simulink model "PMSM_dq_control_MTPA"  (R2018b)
settings: Solver=VariableStepAuto  StartTime=0.0  StopTime=765  FixedStep=1e-5  RelTol=1e-8
InitFcn:
  | I_peak = 230
  | Ke_nom = 0.92
  | Ld_nom = 1.52e-3
  | Lq_nom = 1.54e-3
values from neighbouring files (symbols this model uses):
  B = 0    [Tesla_Initialization.m]    (also in PMSM_EV_init_v2.m; Leaf_Initialization.m)
  J = 0.3    [Tesla_Initialization.m]    (also in PMSM_EV_init_v2.m; Leaf_Initialization.m)
  P = 8    [Tesla_Initialization.m]    (also in PMSM_EV_init_v2.m; Iqbal Husain - Example12_1.m = V.*I; Leaf_Initialization.m)
  radius = 0.447    [Tesla_Initialization.m]    (also in PMSM_EV_init_v2.m = 0.3; Leaf_Initialization.m)
  ratio = 9    [Tesla_Initialization.m]    (also in PMSM_EV_init_v2.m; Leaf_Initialization.m)
  Rs = 0.046    [Tesla_Initialization.m]    (also in PMSM_EV_init_v2.m; Leaf_Initialization.m)
  Tesla_id_axis = [-8.764242E+02	-7.790438E+02	-6.816633E+02	-5.842828E+02	-4.869024E+02	-3.895219E+02	-2.921414E+02	-1.947609E+02	-9.738047E+01	+0.000000E+00]    [Tesla_Initialization.m]
  Tesla_iq_axis = [+0.000000E+00	+9.738047E+01	+1.947609E+02	+2.921414E+02	+3.895219E+02	+4.869024E+02	+5.842828E+02	+6.816633E+02	+7.790438E+02	+8.764242E+02]    [Tesla_Initialization.m]
  Tesla_Ld = [+8.821895E-05	+8.924938E-05	+9.139742E-05	+9.462732E-05	+1.042993E-04	+1.207302E-04	+1.435858E-04	+1.651379E-04	+1.771179E-04	+1.815302E-04    [Tesla_Initialization.m]
  Tesla_Lq = [+2.750008E-04	+2.848007E-04	+2.919706E-04	+2.981362E-04	+3.048757E-04	+3.200995E-04	+3.552424E-04	+3.955550E-04	+4.296280E-04	+4.500669E-04    [Tesla_Initialization.m]
  Tesla_phid = [-9.964313E-02	-8.749389E-02	-7.506085E-02	-6.231998E-02	-4.899731E-02	-3.359246E-02	-1.574417E-02	+5.955898E-03	+2.974036E-02	+5.474011E-02    [Tesla_Initialization.m]
  Tesla_phiq = [+1.577834E-05	+2.291095E-05	+1.626960E-05	+6.018524E-06	+7.523247E-06	+1.073346E-05	+2.148179E-05	+1.486713E-05	+9.491501E-06	-7.613491E-07    [Tesla_Initialization.m]
undefined symbols (not defined in the file or in its folder): A1, B766, HEV_Param
libraries: fl_lib x18, nesl_utility x9, sdl_lib x4

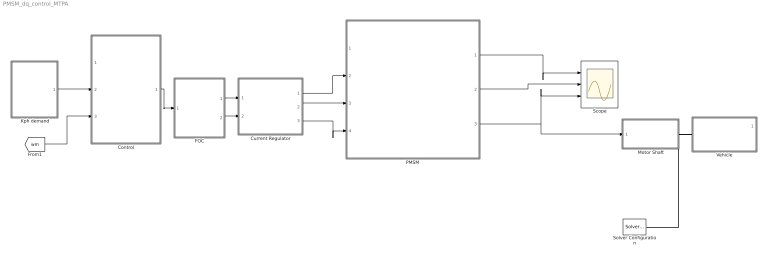
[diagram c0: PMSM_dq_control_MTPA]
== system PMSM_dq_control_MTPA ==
  Control : Subsystem
  Current Regulator : Subsystem
  FOC : Subsystem
  Kph demand : Subsystem
  Motor Shaft : Subsystem
  PMSM : Subsystem
  Scope : Scope  NumInputPorts=3
  Solver Configuration : nesl_utility/Solver Configuration  PhysicalDomain=network_engine_domain  SubClassName=solver  LeftPortType=input  RightPortType=generic  Tones=[]  Harmonics=[]  SimulateNoise=off  Profile=off  UseLocalSampling=off  EnableSwitchedLinearOptims=on  FrequencyDomain=off  UseCCode=off  RelTol=0.001  AbsTol=1e-06  MinStep=1e-09  ToWorkspace=off  RevertToSquareIcSolve=off  NumHomotopyIterations=100  PhasorMode=off  PhasorModeNumHarmonics=1  DoDC=off  ResidualTolerance=1e-09  UseLocalSolver=off  LocalSolverChoice=NE_BACKWARD_EULER_ADVANCER  LocalSolverSampleTime=0.001  DoFixedCost=off  MaxNonlinIter=3  MaxModeIter=2  LinearAlgebra=auto  EquationFormulation=NE_TIME_EF  DelaysMemoryBudget=1024  AutomaticFiltering=on  FilteringTimeConstant=0.001  PartitionStorageMethod=AS_NEEDED  PartitionMemoryBudget=1024
  Vehicle : Subsystem
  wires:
  Current Regulator/1(Va) -> PMSM/2(Va)
  Kph demand/1(Ref omega) -> Control/2(omega_ref)
  PMSM/3(Torque (Nm)) -> Motor Shaft/1(In1), Scope/3
  FOC/2(Id_ref) -> Current Regulator/2(id_ref)
  FOC/1(Iq_ref) -> Current Regulator/1(iq_ref)
  Current Regulator/2(Vb) -> PMSM/3(Vb)
  Current Regulator/3(Vc) -> PMSM/4(Vc)
  PMSM/1(iabc) -> Scope/1
  Control/1(Tref) -> FOC/1(Tref)
  [wm] -> Control/3(omega)
  PMSM/2(wm) -> Scope/2
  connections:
  Vehicle/LConn1 -- Solver Configuration/RConn1 -- Motor Shaft/RConn1

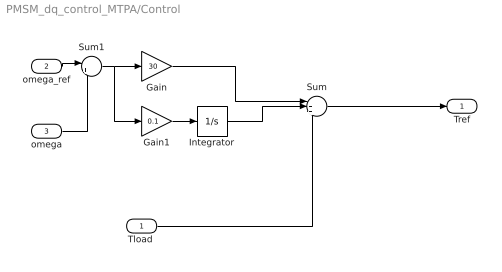
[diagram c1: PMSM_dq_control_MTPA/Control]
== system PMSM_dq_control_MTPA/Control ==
  "Tload " : Inport
  omega_ref : Inport  Port=2
  omega : Inport  Port=3
  Gain : Gain  Gain=30
  Gain1 : Gain  Gain=0.1
  Integrator : Integrator
  Sum : Sum  Inputs=|+++
  Sum1 : Sum  Inputs=|+-
  Tref : Outport
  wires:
  omega_ref/1 -> Sum1/1
  Sum1/1 -> Gain1/1, Gain/1
  omega/1 -> Sum1/2
  Gain1/1 -> Integrator/1
  "Tload "/1 -> Sum/3
  Integrator/1 -> Sum/2
  Gain/1 -> Sum/1
  Sum/1 -> Tref/1

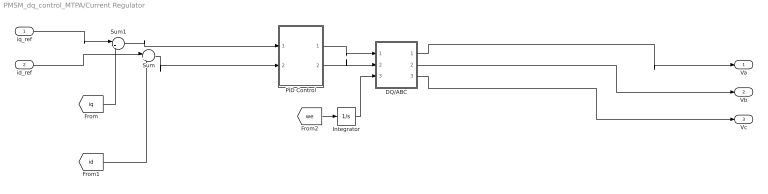
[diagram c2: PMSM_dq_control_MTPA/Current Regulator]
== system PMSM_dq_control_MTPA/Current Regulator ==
  iq_ref : Inport
  id_ref : Inport  Port=2
  DQ/ABC : Subsystem
  Integrator : Integrator
  PID Control : Subsystem
  Sum : Sum  Inputs=|+-
  Sum1 : Sum  Inputs=|+-
  Va : Outport
  Vb : Outport  Port=2
  Vc : Outport  Port=3
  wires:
  [iq] -> Sum1/2
  [id] -> Sum/2
  PID Control/1(Out1) -> DQ/ABC/1(Vq)
  Sum/1 -> PID Control/2(In3)
  PID Control/2(Out2) -> DQ/ABC/2(Vd)
  id_ref/1 -> Sum/1
  [we] -> Integrator/1
  iq_ref/1 -> Sum1/1
  Integrator/1 -> DQ/ABC/3(theta_rf)
  Sum1/1 -> PID Control/1(In1)
  DQ/ABC/1(Va) -> Va/1
  DQ/ABC/2("Vb ") -> Vb/1
  DQ/ABC/3("Vc ") -> Vc/1

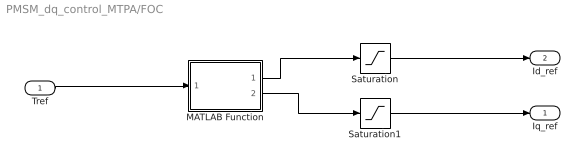
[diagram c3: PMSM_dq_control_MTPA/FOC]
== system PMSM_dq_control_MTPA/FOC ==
  Tref : Inport
  MATLAB Function : MATLAB Function  TreatAsAtomicUnit=on
  Saturation : Saturate  UpperLimit=230  LowerLimit=-230
  Saturation1 : Saturate  UpperLimit=230  LowerLimit=-230
  Iq_ref : Outport
  Id_ref : Outport  Port=2
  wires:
  MATLAB Function/2(iq) -> Saturation1/1
  Saturation/1 -> Id_ref/1
  Saturation1/1 -> Iq_ref/1
  MATLAB Function/1(id) -> Saturation/1
  Tref/1 -> MATLAB Function/1(Te)

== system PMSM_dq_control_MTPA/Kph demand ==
  From Spreadsheet4 : FromSpreadsheet  FileName=Highway_cycle.xlsx  Range=A1:B766  ExtrapolationBeforeFirstDataPoint=Hold first value
  Gain : Gain  Gain=1.6*5/18*ratio/radius
  Ref omega : Outport
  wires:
  From Spreadsheet4/1 -> Gain/1
  Gain/1 -> Ref omega/1

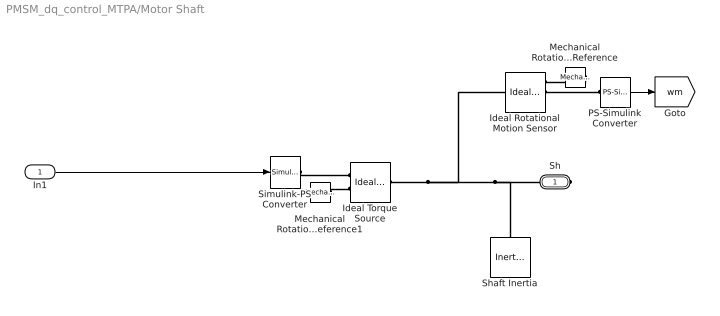
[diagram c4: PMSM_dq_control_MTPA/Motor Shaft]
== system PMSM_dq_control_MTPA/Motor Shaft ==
  In1 : Inport
  Ideal Rotational Motion Sensor : fl_lib/Mechanical/Mechanical Sensors/Ideal Rotational Motion Sensor  offset=0 rad
  Ideal Torque Source : fl_lib/Mechanical/Mechanical Sources/Ideal Torque Source
  Mechanical Rotational Reference : fl_lib/Mechanical/Rotational Elements/Mechanical Rotational Reference
  Mechanical Rotational Reference1 : fl_lib/Mechanical/Rotational Elements/Mechanical Rotational Reference
  PS-Simulink Converter : nesl_utility/PS-Simulink Converter  PhysicalDomain=network_engine_domain  SubClassName=ps_output  LeftPortType=input  RightPortType=output  PseudoPeriodic=off  Frequencies=[]  Unit=rad/s  AffineConversion=off
  Shaft Inertia : fl_lib/Mechanical/Rotational Elements/Inertia  inertia=HEV_Param.Motor.Shaft_Inertia kg*m^2  w_specify=on  w_priority=High  w=0 rad/s  w_nominal_specify=off  w_nominal_unit=rad/s  w_nominal_value=1  t_specify=off  t_priority=High  t=0 N*m  t_nominal_specify=off  t_nominal_unit=N*m  t_nominal_value=1
  Simulink-PS Converter : nesl_utility/Simulink-PS Converter  PhysicalDomain=network_engine_domain  SubClassName=ps_input  LeftPortType=input  RightPortType=output  PseudoPeriodic=off  Frequencies=[]  NoiseDistribution=none  NoiseParameters=[]  Unit=1  AffineConversion=off  FilteringAndDerivatives=zero  SimscapeFilterOrder=1  InputFilterTimeConstant=.001  UdotUserProvided=0
  Sh : PMIOPort  Side=Right
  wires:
  In1/1 -> Simulink-PS Converter/1
  PS-Simulink Converter/1 -> [wm]
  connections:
  Mechanical Rotational Reference1/LConn1 -- Ideal Torque Source/RConn2
  Ideal Torque Source/LConn1 -- Ideal Rotational Motion Sensor/LConn1 -- Shaft Inertia/LConn1 -- Sh/RConn1
  Simulink-PS Converter/RConn1 -- Ideal Torque Source/RConn1
  Mechanical Rotational Reference/LConn1 -- Ideal Rotational Motion Sensor/RConn1
  PS-Simulink Converter/LConn1 -- Ideal Rotational Motion Sensor/RConn2

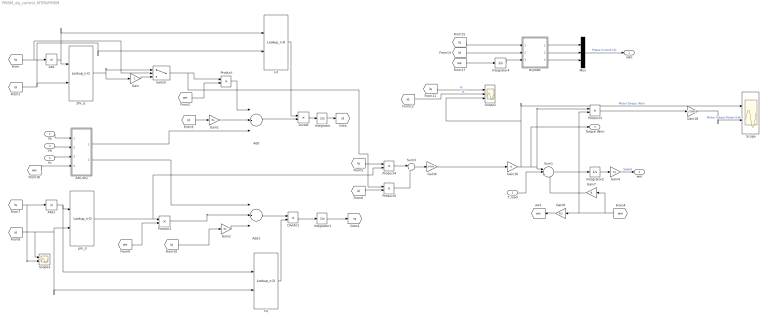
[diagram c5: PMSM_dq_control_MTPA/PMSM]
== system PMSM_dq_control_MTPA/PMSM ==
  T_load : Inport
  Va : Inport  Port=2
  Vb : Inport  Port=3
  Vc : Inport  Port=4
  ABC/DQ : Subsystem
  Abs : Abs
  Abs1 : Abs
  Add : Sum  Inputs=+-+
  Add1 : Sum  Inputs=+--
  DQ/ABC : Subsystem
  Divide : Product  Inputs=/*
  Divide1 : Product  Inputs=*/
  Gain : Gain  Gain=-1
  Gain1 : Gain  Gain=Rs
  Gain16 : Gain
  Gain18 : Gain  Gain=1/1000
  Gain2 : Gain  Gain=Rs
  Gain4 : Gain  Gain=1/J
  Gain6 : Gain  Gain=3*P/4
  Gain7 : Gain  Gain=B
  Gain8 : Gain  Gain=P/2
  Integrator{,1..2,4} (4 alike) : Integrator
  Ld : Lookup_n-D  BreakpointsForDimension1=Tesla_iq_axis  BreakpointsForDimension2=Tesla_id_axis  Table=Tesla_Ld  InternalRulePriority=Speed  RndMeth=Simplest
  Lq : Lookup_n-D  BreakpointsForDimension1=Tesla_iq_axis  BreakpointsForDimension2=Tesla_id_axis  Table=Tesla_Lq  InternalRulePriority=Speed  RndMeth=Simplest
  Mux : Mux  Inputs=3
  Product{,1,3..5} (5 alike) : Product
  Scope : Scope  NumInputPorts=2
  Scope2 : Scope  NumInputPorts=3
  Scope3 : Scope  NumInputPorts=2
  Sum1 : Sum  Inputs=|+--
  Sum3 : Sum  Inputs=|+-
  Switch : Switch  Criteria=u2 > Threshold
  phi_d : Lookup_n-D  BreakpointsForDimension1=Tesla_iq_axis  BreakpointsForDimension2=Tesla_id_axis  Table=Tesla_phid  InternalRulePriority=Speed  RndMeth=Simplest
  phi_q : Lookup_n-D  BreakpointsForDimension1=Tesla_iq_axis  BreakpointsForDimension2=Tesla_id_axis  Table=Tesla_phiq  InternalRulePriority=Speed  RndMeth=Simplest
  iabc : Outport
  wm : Outport  Port=2
  Torque (Nm) : Outport  Port=3
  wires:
  [iq] -> Scope3/2, Abs1/1
  Divide1/1 -> Integrator1/1
  [we] -> ABC/DQ/4(omega_rf)
  [id] -> Scope3/1, Lq/2, phi_d/2
  [id] -> Ld/2, phi_q/2
  Vb/1 -> ABC/DQ/2(Vb)
  Integrator4/1 -> DQ/ABC/3(theta_rf)
  [we] -> Integrator4/1
  [iq] -> DQ/ABC/1(Iq)
  Abs/1 -> Ld/1, phi_q/1
  Gain4/1 -> wm/1  "Speed"
  Divide/1 -> Integrator/1
  Add1/1 -> Divide1/1
  Gain1/1 -> Add/2
  [id] -> DQ/ABC/2(Id)
  Abs1/1 -> Lq/1, phi_d/1
  Integrator2/1 -> Gain4/1
  Ld/1 -> Divide/1
  [we] -> Product/2
  phi_q/1 -> Gain/1, Switch/1
  Product/1 -> Add/1
  Integrator1/1 -> [iq]
  T_load/1 -> Sum1/2
  [iq] -> Switch/2, Abs/1
  Add/1 -> Divide/2
  Sum1/1 -> Integrator2/1
  [we] -> Product1/2
  Va/1 -> ABC/DQ/1(Va)
  Integrator/1 -> [id]
  Gain/1 -> Switch/3
  Mux/1 -> iabc/1  "Phase Current (A)"
  Gain2/1 -> Add1/3
  DQ/ABC/2("Ib ") -> Mux/2
  DQ/ABC/3("Ic ") -> Mux/3
  Gain7/1 -> Sum1/3
  Gain8/1 -> [we]
  Gain16/1 -> Torque (Nm)/1, Product3/1, Sum1/1, Scope/1, Scope2/3  "Motor Torque (Nm)"
  [iq] -> Scope2/1  "iq"
  Product3/1 -> Gain18/1
  Gain18/1 -> Scope/2  "Motor Output Power (kW)"
  Vc/1 -> ABC/DQ/3(Vc)
  ABC/DQ/2("q ") -> Add1/1
  [id] -> Gain1/1
  ABC/DQ/1(d) -> Add/3
  [iq] -> Gain2/1
  DQ/ABC/1(Ia) -> Mux/1
  Product1/1 -> Add1/2
  [wm] -> Gain8/1, Product3/2, Gain7/1
  [iq] -> Product4/1
  Switch/1 -> Product5/1, Product/1
  Gain6/1 -> Gain16/1
  Product5/1 -> Sum3/2
  Sum3/1 -> Gain6/1
  phi_d/1 -> Product4/2, Product1/1
  [id] -> Product5/2
  Product4/1 -> Sum3/1
  Lq/1 -> Divide1/2
  [id] -> Scope2/2  "id"

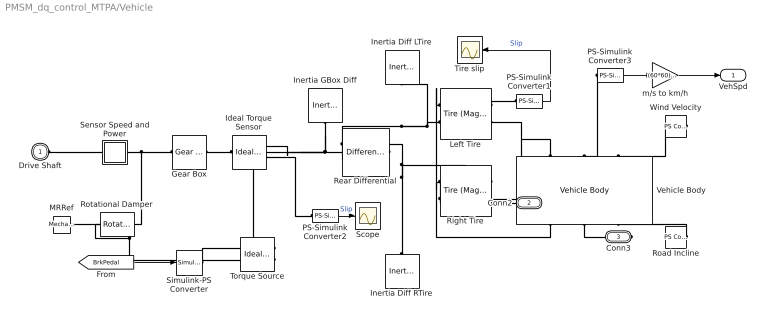
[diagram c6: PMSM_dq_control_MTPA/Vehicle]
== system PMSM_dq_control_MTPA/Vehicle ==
  Gear Box : fl_lib/Mechanical/Mechanisms/Gear Box  ratio=HEV_Param.Vehicle.Engine_Vehicle_Gear_Ratio  t_in_specify=off  t_in_priority=High  t_in=0 N*m  t_in_nominal_specify=off  t_in_nominal_unit=N*m  t_in_nominal_value=1  t_out_specify=off  t_out_priority=High  t_out=0 N*m  t_out_nominal_specify=off  t_out_nominal_unit=N*m  t_out_nominal_value=1
  Ideal Torque Sensor : fl_lib/Mechanical/Mechanical Sensors/Ideal Torque Sensor
  Inertia Diff LTire : fl_lib/Mechanical/Rotational Elements/Inertia  inertia=HEV_Param.Vehicle.Wheel_Inertia*2 kg*m^2  w_specify=on  w_priority=High  w=0 rad/s  w_nominal_specify=off  w_nominal_unit=rad/s  w_nominal_value=1  t_specify=off  t_priority=High  t=0 N*m  t_nominal_specify=off  t_nominal_unit=N*m  t_nominal_value=1
  Inertia Diff RTire : fl_lib/Mechanical/Rotational Elements/Inertia  inertia=HEV_Param.Vehicle.Wheel_Inertia*2 kg*m^2  w_specify=on  w_priority=High  w=0 rad/s  w_nominal_specify=off  w_nominal_unit=rad/s  w_nominal_value=1  t_specify=off  t_priority=High  t=0 N*m  t_nominal_specify=off  t_nominal_unit=N*m  t_nominal_value=1
  Inertia GBox Diff : fl_lib/Mechanical/Rotational Elements/Inertia  inertia=HEV_Param.Vehicle.Trans.Inertia kg*m^2  w_specify=on  w_priority=High  w=0 rad/s  w_nominal_specify=off  w_nominal_unit=rad/s  w_nominal_value=1  t_specify=off  t_priority=High  t=0 N*m  t_nominal_specify=off  t_nominal_unit=N*m  t_nominal_value=1
  Left Tire : sdl_lib/Tires & Vehicles/Tire (Magic Formula)  parameterization=1  F_z1=HEV_Param.Vehicle.Tire.Rated_Vertical_Load N  F_x1=HEV_Param.Vehicle.Tire.Rated_Peak_Long_Force N  kappa1=HEV_Param.Vehicle.Tire.Slip_At_Peak_Force  B_m=10  C_m=1.9  D_m=1  E_m=0.97  fz0=4e+3 N  p_Cx=1.685  p_Dx=[ 1.21 -0.037 ]  p_Ex=[ 0.344 0.095 -0.02 0 ]  p_Kx=[ 21.51 -0.163 0.245 ]  p_Hx=[ -0.002 0.002 ]  p_Vx=[ 0 0 ]  v_tr_thr=0.1 m/s  r_e=HEV_Param.Vehicle.Tire_Radius m  model_compliance=0  stiffness=1e+6 N/m  damping=1000 N/(m/s)  model_inertia=1  inertia=1e-2 kg*m^2  initial_velocity=0 rpm  model_resistance=1  resistance_model=1  coeff=0.015  p_tire=250e3 Pa  alpha=-0.003  beta=0.97  coeff_a=84e-4  coeff_b=6.2e-4 s/m  coeff_c=1.6e-4 s^2/m^2  v_thr=1e-3 m/s
  MRRef : fl_lib/Mechanical/Rotational Elements/Mechanical Rotational Reference
  PS-Simulink Converter1 : nesl_utility/PS-Simulink Converter  PhysicalDomain=network_engine_domain  SubClassName=ps_output  LeftPortType=input  RightPortType=output  PseudoPeriodic=off  Frequencies=[]  Unit=1  AffineConversion=off
  PS-Simulink Converter2 : nesl_utility/PS-Simulink Converter  PhysicalDomain=network_engine_domain  SubClassName=ps_output  LeftPortType=input  RightPortType=output  PseudoPeriodic=off  Frequencies=[]  Unit=1  AffineConversion=off
  PS-Simulink Converter3 : nesl_utility/PS-Simulink Converter  PhysicalDomain=network_engine_domain  SubClassName=ps_output  LeftPortType=input  RightPortType=output  PseudoPeriodic=off  Frequencies=[]  Unit=m/s  AffineConversion=off
  Rear Differential : sdl_lib/Gears/Differential  driveshaft_location=2  cd_ratio=1  friction_model=1  efficiency=[ 0.85 0.92 ]  mu_visc=[ 0 0 ] N*m/(rad/s)  pwr_thr=[ 0.001 0.001 ] W  carrier_inertia=0 kg*m^2  planet_inertia=0 kg*m^2  temperature_TLU=[ 280 300 320 ] K  efficiency_ss_TLU=[ 0.95 0.9 0.85 ]  efficiency_cd_TLU=[ 0.95 0.9 0.85 ]  thermal_mass=50 J/K  T_init=300 K
  Right Tire : sdl_lib/Tires & Vehicles/Tire (Magic Formula)  parameterization=1  F_z1=HEV_Param.Vehicle.Tire.Rated_Vertical_Load N  F_x1=HEV_Param.Vehicle.Tire.Rated_Peak_Long_Force N  kappa1=HEV_Param.Vehicle.Tire.Slip_At_Peak_Force  B_m=10  C_m=1.9  D_m=1  E_m=0.97  fz0=4e+3 N  p_Cx=1.685  p_Dx=[ 1.21 -0.037 ]  p_Ex=[ 0.344 0.095 -0.02 0 ]  p_Kx=[ 21.51 -0.163 0.245 ]  p_Hx=[ -0.002 0.002 ]  p_Vx=[ 0 0 ]  v_tr_thr=0.1 m/s  r_e=HEV_Param.Vehicle.Tire_Radius m  model_compliance=0  stiffness=1e+6 N/m  damping=1000 N/(m/s)  model_inertia=1  inertia=1e-2 kg*m^2  initial_velocity=0 rpm  model_resistance=1  resistance_model=1  coeff=0.015  p_tire=250e3 Pa  alpha=-0.003  beta=0.97  coeff_a=84e-4  coeff_b=6.2e-4 s/m  coeff_c=1.6e-4 s^2/m^2  v_thr=1e-3 m/s
  Road Incline : fl_lib/Physical Signals/Sources/PS Constant  constant=HEV_Param.Vehicle.Incline
  Rotational Damper : fl_lib/Mechanical/Rotational Elements/Rotational Damper  D=HEV_Param.Vehicle.Trans.Friction N*m/(rad/s)  w_specify=off  w_priority=High  w=0 rad/s  w_nominal_specify=off  w_nominal_unit=rad/s  w_nominal_value=1  t_specify=off  t_priority=High  t=0 N*m  t_nominal_specify=off  t_nominal_unit=N*m  t_nominal_value=1
  Scope : Scope
  Sensor Speed and Power : Subsystem
  Simulink-PS Converter : nesl_utility/Simulink-PS Converter  PhysicalDomain=network_engine_domain  SubClassName=ps_input  LeftPortType=input  RightPortType=output  PseudoPeriodic=off  Frequencies=[]  NoiseDistribution=none  NoiseParameters=[]  Unit=1  AffineConversion=off  FilteringAndDerivatives=zero  SimscapeFilterOrder=1  InputFilterTimeConstant=0.001  UdotUserProvided=1
  Tire slip : Scope
  Torque Source : fl_lib/Mechanical/Mechanical Sources/Ideal Torque Source
  Vehicle Body : sdl_lib/Tires & Vehicles/Vehicle Body  mass=HEV_Param.Vehicle.Mass kg  n_w=2  x_f=HEV_Param.Vehicle.Distance_CG_FrontAxle m  x_r=HEV_Param.Vehicle.Distance_CG_RearAxle m  y_c=HEV_Param.Vehicle.Distance_CG_Ground m  model_pitch=0  inertia=4000 kg*m^2  suspension_model=1  k_f=1e4 N/m  b_f=1e4 N/(m/s)  k_r=1e4 N/m  b_r=1e4 N/(m/s)  k_f_TLU=[-2000, -1000, 0, 1000, 2000] N  x_f_TLU=[-.4, -.2, 0, .2, .4] m  b_f_TLU=[-200, -100, 0, 100, 200] N  v_f_TLU=[-4, -2, 0, 2, 4] m/s  k_r_TLU=[-2000, -1000, 0, 1000, 2000] N  x_r_TLU=[-.4, -.2, 0, .2, .4] m  b_r_TLU=[-200, -100, 0, 100, 200] N  v_r_TLU=[-4, -2, 0, 2, 4] m/s  interp_method=simscape.enum.interpolation.linear  extrap_method=simscape.enum.extrapolation.linear  model_hardstop=0  upper_bound_f=.25 m  lower_bound_f=-.25 m  stop_k_f=1e6 N/m  stop_b_f=150 N/(m/s)  upper_bound_r=.25 m  lower_bound_r=-.25 m  stop_k_r=1e6 N/m  stop_b_r=150 N/(m/s)  initial_pitch=0 rad  initial_pitch_rate=0 rad/s  g=9.81 m/s^2  liftoff_warning=0  area=HEV_Param.Vehicle.Frontal_Area m^2  Cd=HEV_Param.Vehicle.Aero_Drag_Coeff  rho=1.18 kg/m^3  v_specify=on  v_priority=High  v=0 m/s  v_nominal_specify=off  v_nominal_unit=m/s  v_nominal_value=1
  Wind Velocity : fl_lib/Physical Signals/Sources/PS Constant  constant=0
  m/s to km/h : Gain  Gain=(60*60)/1000
  Drive Shaft : PMIOPort  Side=Left
  Conn2 : PMIOPort  Port=2  Side=Right
  Conn3 : PMIOPort  Port=3  Side=Right
  VehSpd : Outport
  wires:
  PS-Simulink Converter2/1 -> Scope/1  "Slip"
  PS-Simulink Converter3/1 -> m/s to km/h/1
  [BrkPedal] -> Simulink-PS Converter/1
  PS-Simulink Converter1/1 -> Tire slip/1  "Slip"
  m/s to km/h/1 -> VehSpd/1
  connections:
  Drive Shaft/RConn1 -- Sensor Speed and Power/LConn1
  Vehicle Body/LConn1 -- Right Tire/RConn2 -- Left Tire/RConn2
  Sensor Speed and Power/RConn1 -- Rotational Damper/LConn1 -- Gear Box/LConn1
  Torque Source/RConn2 -- Rotational Damper/RConn1 -- MRRef/LConn1
  Road Incline/RConn1 -- Vehicle Body/RConn3
  Inertia GBox Diff/LConn1 -- Rear Differential/LConn1 -- Torque Source/LConn1 -- Ideal Torque Sensor/RConn1
  Left Tire/RConn1 -- PS-Simulink Converter1/LConn1
  Wind Velocity/RConn1 -- Vehicle Body/LConn3
  Simulink-PS Converter/RConn1 -- Torque Source/RConn1
  PS-Simulink Converter2/LConn1 -- Ideal Torque Sensor/RConn2
  PS-Simulink Converter3/LConn1 -- Vehicle Body/LConn2
  Ideal Torque Sensor/LConn1 -- Gear Box/RConn1
  Vehicle Body/RConn1 -- Right Tire/LConn1 -- Left Tire/LConn1
  Vehicle Body/RConn2 -- Conn3/RConn1
  Left Tire/LConn2 -- Rear Differential/RConn2 -- Inertia Diff LTire/LConn1
  Right Tire/RConn1 -- Conn2/RConn1
  Rear Differential/RConn1 -- Right Tire/LConn2 -- Inertia Diff RTire/LConn1

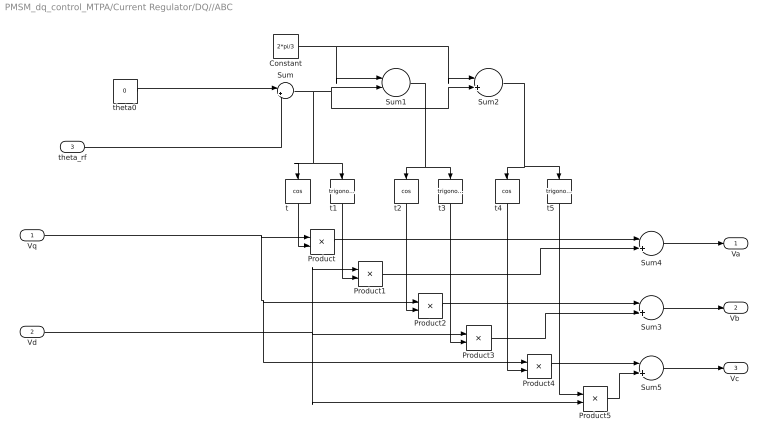
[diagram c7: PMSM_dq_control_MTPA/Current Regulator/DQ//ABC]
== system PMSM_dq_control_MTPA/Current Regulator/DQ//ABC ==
  Vq : Inport
  Vd : Inport  Port=2
  theta_rf : Inport  Port=3
  Constant : Constant  Value=2*pi/3
  Product{,1..5} (6 alike) : Product
  Sum{,2..5} (5 alike) : Sum  Inputs=|++
  Sum1 : Sum  Inputs=|-+
  t : Trigonometry  Operator=cos
  t1 : Trigonometry
  t2 : Trigonometry  Operator=cos
  t3 : Trigonometry
  t4 : Trigonometry  Operator=cos
  t5 : Trigonometry
  theta0 : Constant  Value=0
  Va : Outport
  "Vb " : Outport  Port=2
  "Vc " : Outport  Port=3
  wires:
  theta0/1 -> Sum/1
  Sum/1 -> t1/1, t/1, Sum2/2, Sum1/2
  Sum2/1 -> t5/1, t4/1
  Sum1/1 -> t2/1, t3/1
  t/1 -> Product/2
  Constant/1 -> Sum1/1, Sum2/1
  Product3/1 -> Sum3/2
  t1/1 -> Product1/2
  t3/1 -> Product3/2
  t2/1 -> Product2/2
  Sum4/1 -> Va/1
  Sum3/1 -> "Vb "/1
  theta_rf/1 -> Sum/2
  Vd/1 -> Product5/2, Product1/1, Product3/1
  Product/1 -> Sum4/1
  Product1/1 -> Sum4/2
  Product2/1 -> Sum3/1
  Vq/1 -> Product4/1, Product2/1, Product/1
  t4/1 -> Product4/2
  t5/1 -> Product5/1
  Product4/1 -> Sum5/1
  Product5/1 -> Sum5/2
  Sum5/1 -> "Vc "/1

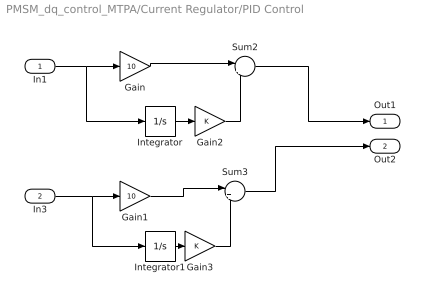
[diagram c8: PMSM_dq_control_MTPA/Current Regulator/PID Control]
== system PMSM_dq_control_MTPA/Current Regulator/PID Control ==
  In1 : Inport
  In3 : Inport  Port=2
  Gain : Gain  Gain=10
  Gain1 : Gain  Gain=10
  Gain2 : Gain
  Gain3 : Gain
  Integrator : Integrator
  Integrator1 : Integrator
  Sum2 : Sum  Inputs=|++
  Sum3 : Sum  Inputs=|++
  Out1 : Outport
  Out2 : Outport  Port=2
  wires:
  Integrator1/1 -> Gain3/1
  Gain1/1 -> Sum3/1
  Gain2/1 -> Sum2/2
  Gain/1 -> Sum2/1
  In1/1 -> Integrator/1, Gain/1
  Sum2/1 -> Out1/1
  In3/1 -> Integrator1/1, Gain1/1
  Integrator/1 -> Gain2/1
  Gain3/1 -> Sum3/2
  Sum3/1 -> Out2/1

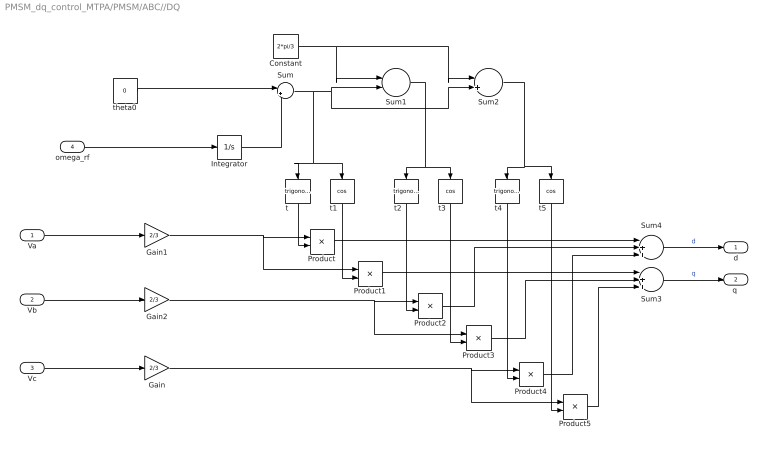
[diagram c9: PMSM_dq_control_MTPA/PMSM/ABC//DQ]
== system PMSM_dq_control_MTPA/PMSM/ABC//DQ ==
  Va : Inport
  Vb : Inport  Port=2
  Vc : Inport  Port=3
  omega_rf : Inport  Port=4
  Constant : Constant  Value=2*pi/3
  Gain : Gain  Gain=2/3
  Gain1 : Gain  Gain=2/3
  Gain2 : Gain  Gain=2/3
  Integrator : Integrator
  Product{,1..5} (6 alike) : Product
  Sum : Sum  Inputs=|++
  Sum1 : Sum  Inputs=|-+
  Sum2 : Sum  Inputs=|++
  Sum3 : Sum  Inputs=|+++
  Sum4 : Sum  Inputs=|+++
  t : Trigonometry
  t1 : Trigonometry  Operator=cos
  t2 : Trigonometry
  t3 : Trigonometry  Operator=cos
  t4 : Trigonometry
  t5 : Trigonometry  Operator=cos
  theta0 : Constant  Value=0
  d : Outport
  "q " : Outport  Port=2
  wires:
  theta0/1 -> Sum/1
  Sum/1 -> t1/1, t/1, Sum2/2, Sum1/2
  Sum2/1 -> t5/1, t4/1
  Integrator/1 -> Sum/2
  t4/1 -> Product4/2
  Sum1/1 -> t2/1, t3/1
  Product/1 -> Sum4/1
  t/1 -> Product/2
  Va/1 -> Gain1/1
  Constant/1 -> Sum1/1, Sum2/1
  Vc/1 -> Gain/1
  Product3/1 -> Sum3/2
  Gain2/1 -> Product3/1, Product2/1
  t5/1 -> Product5/2
  t1/1 -> Product1/2
  Gain/1 -> Product5/1, Product4/1
  Product1/1 -> Sum3/1
  Gain1/1 -> Product1/1, Product/1
  Product5/1 -> Sum3/3
  Product2/1 -> Sum4/2
  Product4/1 -> Sum4/3
  Vb/1 -> Gain2/1
  t3/1 -> Product3/2
  t2/1 -> Product2/2
  Sum4/1 -> d/1  "d"
  Sum3/1 -> "q "/1  "q"
  omega_rf/1 -> Integrator/1

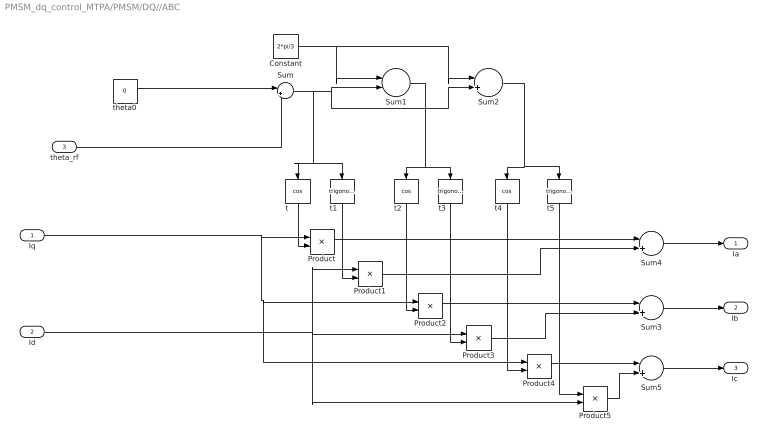
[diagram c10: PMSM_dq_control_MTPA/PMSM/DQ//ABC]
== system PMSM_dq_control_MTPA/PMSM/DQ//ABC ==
  Iq : Inport
  Id : Inport  Port=2
  theta_rf : Inport  Port=3
  Constant : Constant  Value=2*pi/3
  Product{,1..5} (6 alike) : Product
  Sum{,2..5} (5 alike) : Sum  Inputs=|++
  Sum1 : Sum  Inputs=|-+
  t : Trigonometry  Operator=cos
  t1 : Trigonometry
  t2 : Trigonometry  Operator=cos
  t3 : Trigonometry
  t4 : Trigonometry  Operator=cos
  t5 : Trigonometry
  theta0 : Constant  Value=0
  Ia : Outport
  "Ib " : Outport  Port=2
  "Ic " : Outport  Port=3
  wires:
  theta0/1 -> Sum/1
  Sum/1 -> t1/1, t/1, Sum2/2, Sum1/2
  Sum2/1 -> t5/1, t4/1
  Sum1/1 -> t2/1, t3/1
  t/1 -> Product/2
  Constant/1 -> Sum1/1, Sum2/1
  Product3/1 -> Sum3/2
  t1/1 -> Product1/2
  t3/1 -> Product3/2
  t2/1 -> Product2/2
  Sum4/1 -> Ia/1
  Sum3/1 -> "Ib "/1
  theta_rf/1 -> Sum/2
  Id/1 -> Product5/2, Product1/1, Product3/1
  Product/1 -> Sum4/1
  Product1/1 -> Sum4/2
  Product2/1 -> Sum3/1
  Iq/1 -> Product4/1, Product2/1, Product/1
  t4/1 -> Product4/2
  t5/1 -> Product5/1
  Product4/1 -> Sum5/1
  Product5/1 -> Sum5/2
  Sum5/1 -> "Ic "/1

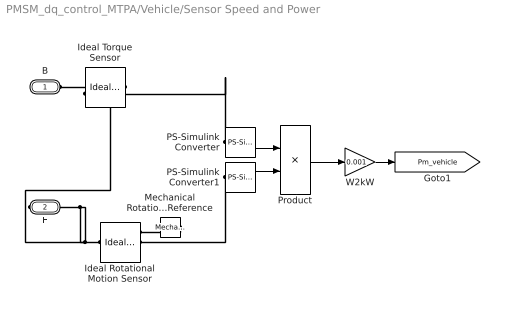
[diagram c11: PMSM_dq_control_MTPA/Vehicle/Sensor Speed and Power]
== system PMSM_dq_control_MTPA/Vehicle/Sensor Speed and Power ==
  Ideal Rotational Motion Sensor : fl_lib/Mechanical/Mechanical Sensors/Ideal Rotational Motion Sensor  offset=0 rad
  Ideal Torque Sensor : fl_lib/Mechanical/Mechanical Sensors/Ideal Torque Sensor
  Mechanical Rotational Reference : fl_lib/Mechanical/Rotational Elements/Mechanical Rotational Reference
  PS-Simulink Converter : nesl_utility/PS-Simulink Converter  PhysicalDomain=network_engine_domain  SubClassName=ps_output  LeftPortType=input  RightPortType=output  PseudoPeriodic=off  Frequencies=[]  Unit=N*m  AffineConversion=off
  PS-Simulink Converter1 : nesl_utility/PS-Simulink Converter  PhysicalDomain=network_engine_domain  SubClassName=ps_output  LeftPortType=input  RightPortType=output  PseudoPeriodic=off  Frequencies=[]  Unit=rad/s  AffineConversion=off
  Product : Product
  W2kW : Gain  Gain=0.001
  B : PMIOPort  Side=Left
  F : PMIOPort  Port=2  Side=Right
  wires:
  W2kW/1 -> [Pm_vehicle]
  Product/1 -> W2kW/1
  PS-Simulink Converter/1 -> Product/1
  PS-Simulink Converter1/1 -> Product/2
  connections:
  Mechanical Rotational Reference/LConn1 -- Ideal Rotational Motion Sensor/RConn1
  Ideal Rotational Motion Sensor/LConn1 -- F/RConn1 -- Ideal Torque Sensor/RConn1
  B/RConn1 -- Ideal Torque Sensor/LConn1
  PS-Simulink Converter/LConn1 -- Ideal Torque Sensor/RConn2
  PS-Simulink Converter1/LConn1 -- Ideal Rotational Motion Sensor/RConn2

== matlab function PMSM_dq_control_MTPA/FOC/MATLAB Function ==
function [id,iq]= fcn(Te)
lambda=0.06;
Ld=0.42e-3;
Lq=0.52e-3;
P=8;
iqp=[1 0 0 4*Te*lambda/(3*P*(Ld-Lq)^2) -(4*Te/(3*P*(Ld-Lq)))^2];
iq=real(min((roots(iqp))));
if Te~=0
   id=4*Te/(3*P*(Ld-Lq)*(iq))-lambda/(Ld-Lq);
else
   id=0;
end
end
